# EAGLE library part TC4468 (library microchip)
Logic-Input CMOS Quad Drivers Source: TC 4469-MOSFET-DRIVER.pdf
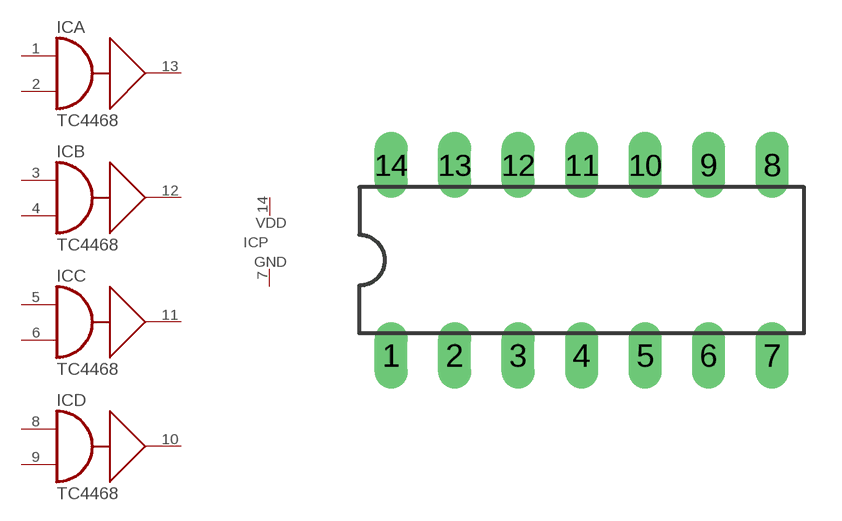
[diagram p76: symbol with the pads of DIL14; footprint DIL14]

Designator prefix IC; gates A=TC4468 B=TC4468 C=TC4468 D=TC4468 P=VDD-GND

## TC4468DP (MF: MICROCHIP; MPN: TC4468CPD; OC_FARNELL: 1557406; OC_NEWARK: 54K2859)  [DIL14]
1  A:A  in
2  A:B  in
3  B:A  in
4  B:B  in
5  C:A  in
6  C:B  in
7  P:GND  pwr
8  D:A  in
9  D:B  in
10  D:Y  out
11  C:Y  out
12  B:Y  out
13  A:Y  out
14  P:VDD  pwr

## TC4468JD (OC_FARNELL: unknown; OC_NEWARK: unknown)  [DIL14]
Pads as for DIL14

## Footprint DIL14 (pad centres in mm)
Dual In Line Package
drill 0.813 long: 1 -7.62,-3.81; 2 -5.08,-3.81; 3 -2.54,-3.81; 4 0,-3.81; 5 2.54,-3.81; 6 5.08,-3.81; 7 7.62,-3.81; 8 7.62,3.81; 9 5.08,3.81; 10 2.54,3.81; 11 0,3.81; 12 -2.54,3.81; 13 -5.08,3.81; 14 -7.62,3.81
